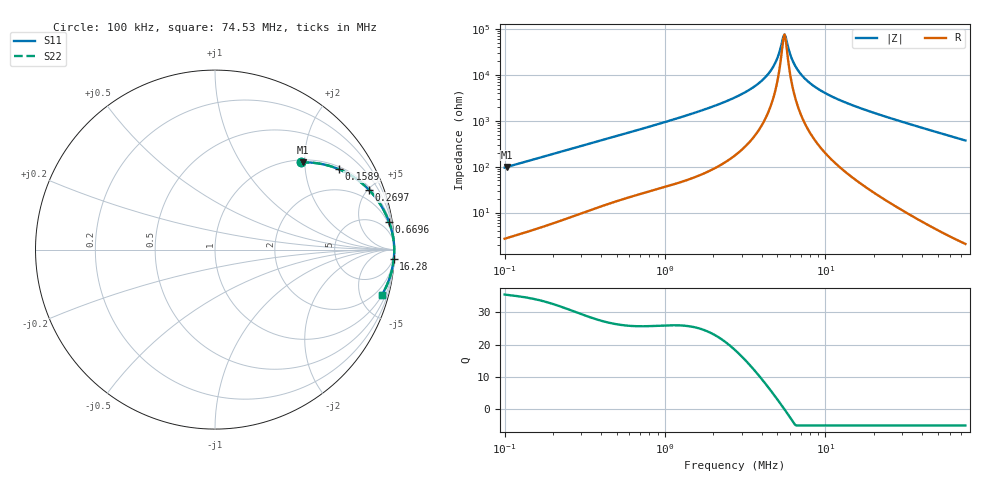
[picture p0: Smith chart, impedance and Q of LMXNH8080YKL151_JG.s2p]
! LMXNH8080YKL151_JG  S-PARAMETER MODEL  ( Standard Model )
! Model Generated by TAIYO YUDEN Corporation (https://www.yuden.co.jp/en/)
! Version 1.0
! TAIYO YUDEN Control No. 20250523
! Copyright(c) 2025 TAIYO YUDEN CO.,LTD. All Rights Reserved.
! Product Description (link to TY-COMPAS)
! https://ds.yuden.co.jp/TYCOMPAS/or/detail?pn=LMXNH8080YKL151MJG&u=M
! Products Name : Inductors
! Characteristics :
!  Inductance : 150 [uH] , SRF(min) : 5.0 [MHz] , DC Resistance(max) : 0.546 [Ohm]
!  Rated Current : Saturation  900 [mA] , Temp Rise  800 [mA] (40 [degC])
!  Case Size : 8.0 x 8.0 / 0.315 x 0.315 [mm/inch] , Thickness : 4.0 / 0.157 [mm/inch]
!  (Conditions: Temperature = 25 [degC] , DC Bias Current = 0 [A])
! External Node Assignments :
!  1  o---GGG---o  2
! GND o---------o GND
! Frequency Range : 0.1MHz  -  74.526194MHz  [ 402 STEP ]
# MHz S RI R 50
! Freq[MHz].  S11 Real  S11 Imag  S21 Real  S21 Imag  S12 Real  S12 Imag  S22 Real  S22 Imag
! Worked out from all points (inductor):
!   401 points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, 100 kHz to 74.53 MHz, reference 50 ohm
!   read as one part in series: L = 151 uH near 103.4 kHz
!   highest Q = 35.4 at 103.4 kHz (marker M1), where L = 151 uH
!   self-resonance near 5.467 MHz
!   S11 on the Smith chart (normalised r, x): 100 kHz: 1.05, +1.90; 158.9 kHz: 1.09, +3.01; 269.7 kHz: 1.17, +5.06; 669.6 kHz: 1, +12; 16.28 MHz: 2, -38; 74.53 MHz: 1.04, -7.43
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0.1  0.4764 0.4855  0.5236 -0.4855  0.5236 -0.4855  0.4764 0.4855
0.103362  0.4922 0.486  0.5078 -0.486  0.5078 -0.486  0.4922 0.486
0.158877  0.6881 0.4488  0.3119 -0.4488  0.3119 -0.4488  0.6881 0.4488
0.269679  0.857 0.3339  0.143 -0.3339  0.143 -0.3339  0.857 0.3339
0.302769  0.8814 0.3067  0.1186 -0.3067  0.1186 -0.3067  0.8814 0.3067
0.669559  0.9691 0.1547  0.0309 -0.1547  0.0309 -0.1547  0.9691 0.1547
0.916692  0.9822 0.1142  0.0178 -0.1142  0.0178 -0.1142  0.9822 0.1142
2.729949  0.9974 0.0309  0.00264 -0.0309  0.00264 -0.0309  0.9974 0.0309
3.615993  0.9982 0.0177  0.00179 -0.0177  0.00179 -0.0177  0.9982 0.0177
4.337266  0.9985 0.01  0.00149 -0.01  0.00149 -0.01  0.9985 0.01
4.869468  0.9986 0.00527  0.00138 -0.00527  0.00138 -0.00527  0.9986 0.00527
5.377323  0.9987 0.00127  0.00133 -0.00127  0.00133 -0.00127  0.9987 0.00127
5.558117  0.9987 -5.52e-05  0.00132 5.52e-05  0.00132 5.52e-05  0.9987 -5.52e-05
5.744989  0.9987 -0.00138  0.00131 0.00138  0.00131 0.00138  0.9987 -0.00138
6.137794  0.9987 -0.00405  0.00131 0.00405  0.00131 0.00405  0.9987 -0.00405
6.557456  0.9987 -0.00673  0.00133 0.00673  0.00133 0.00673  0.9987 -0.00673
7.241358  0.9986 -0.0108  0.00138 0.0108  0.00138 0.0108  0.9986 -0.0108
8.265445  0.9985 -0.0164  0.00152 0.0164  0.00152 0.0164  0.9985 -0.0164
10.94811  0.9979 -0.0294  0.0021 0.0294  0.0021 0.0294  0.9979 -0.0294
16.28088  0.9961 -0.052  0.00393 0.052  0.00393 0.052  0.9961 -0.052
25.02522  0.9914 -0.0855  0.00861 0.0855  0.00861 0.0855  0.9914 -0.0855
74.52619  0.9313 -0.2502  0.0687 0.2502  0.0687 0.2502  0.9313 -0.2502
